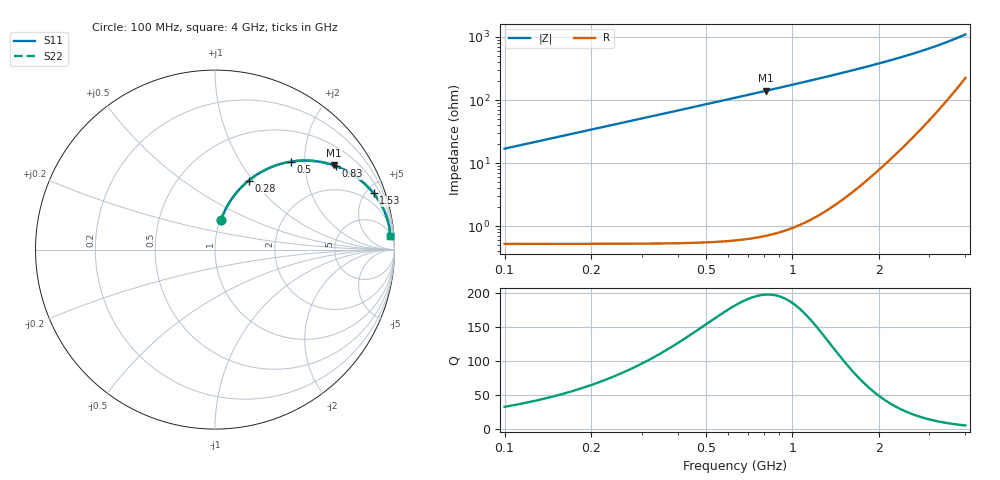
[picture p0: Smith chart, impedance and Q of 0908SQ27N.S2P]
! Coilcraft 0908SQ-27N Air Core Inductor
! 07 March 2008
# MHZ S MA R 50
!Freq  MagS11  AngS11  MagS21  AngS21  MagS12  AngS12  MagS22  AngS22
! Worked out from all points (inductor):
!   391 points, 100 MHz to 4 GHz, reference 50 ohm
!   read as one part in series: L = 27.1 nH near 110 MHz
!   highest Q = 198 at 810 MHz (marker M1), where L = 27.5 nH
!   S11 on the Smith chart (normalised r, x): 100 MHz: 1.01, +0.34; 280 MHz: 1.01, +0.95; 500 MHz: 1.01, +1.71; 830 MHz: 1.02, +2.88; 1.53 GHz: 1.08, +5.61; 4 GHz: 7, +24
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100  0.1666 78.6  0.9809 -9.6  0.9809 -9.6  0.1666 78.6
120  0.1987 77.0  0.9749 -11.5  0.9749 -11.5  0.1987 77.0
140  0.2302 75.4  0.968 -13.3  0.968 -13.3  0.2302 75.4
180  0.2911 72.1  0.9517 -17.0  0.9517 -17.0  0.2911 72.1
230  0.3625 67.9  0.9271 -21.3  0.9271 -21.3  0.3625 67.9
280  0.4282 64.0  0.8989 -25.4  0.8989 -25.4  0.4282 64.0
330  0.4878 60.2  0.8683 -29.3  0.8683 -29.3  0.4879 60.2
380  0.5415 56.7  0.8362 -32.9  0.8362 -32.9  0.5415 56.7
500  0.6475 49.2  0.7578 -40.4  0.7578 -40.4  0.6476 49.2
620  0.7265 43.0  0.6831 -46.7  0.6831 -46.7  0.7265 43.0
750  0.789 37.5  0.6104 -52.2  0.6104 -52.2  0.789 37.5
810  0.8117 35.3  0.58 -54.4  0.58 -54.4  0.8117 35.3
830  0.8186 34.6  0.5703 -55.1  0.5703 -55.1  0.8186 34.6
950  0.8536 30.9  0.5165 -58.8  0.5165 -58.8  0.8536 30.9
1090  0.8839 27.4  0.4626 -62.3  0.4626 -62.3  0.8839 27.4
1240  0.9076 24.2  0.4135 -65.4  0.4135 -65.4  0.9077 24.2
1400  0.9261 21.4  0.3694 -68.1  0.3694 -68.1  0.9261 21.4
1530  0.9375 19.5  0.3385 -69.9  0.3385 -69.9  0.9375 19.5
2050  0.9637 13.9  0.2465 -74.8  0.2465 -74.8  0.9637 13.9
2700  0.976 9.5  0.1732 -77.6  0.1732 -77.6  0.976 9.5
3350  0.979 6.5  0.1242 -77.3  0.1242 -77.3  0.9791 6.5
4000  0.9778 4.3  0.08947 -73.8  0.08947 -73.8  0.9778 4.3
